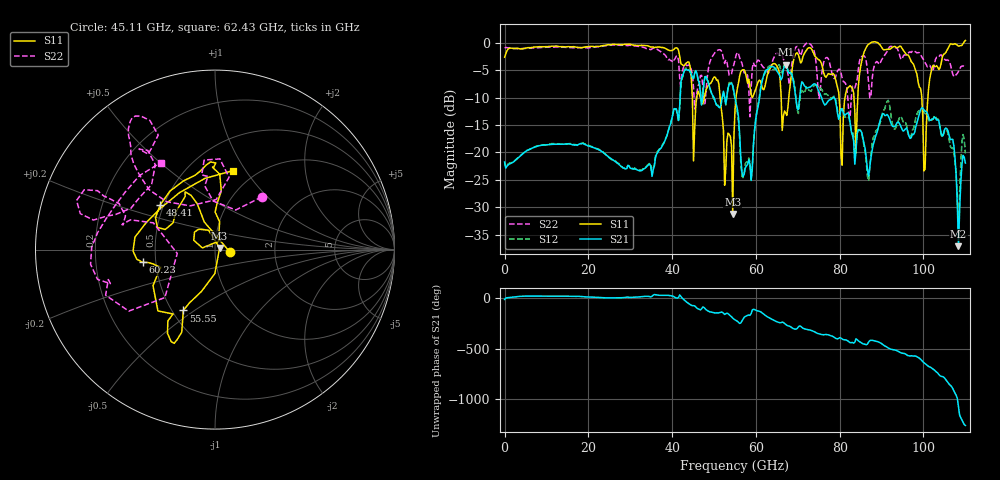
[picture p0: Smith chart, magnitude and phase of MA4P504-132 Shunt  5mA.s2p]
!Keysight Technologies,N5247B,US61255204,A.15.70.20
!Date: Friday, October 21, 2022 14:57:07
!Correction: S11(C  4-Port  )
!S31(C  4-Port  )
!S13(C  4-Port  )
!S33(C  4-Port  )
!S2P File: Measurements: S11, S31, S13, S33:
# Hz S  dB  R 50
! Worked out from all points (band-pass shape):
!   401 points, 10 MHz to 110 GHz, reference 50 ohm
!   highest |S21| = -3.97 dB at 67.1 GHz (marker M1); lowest = -37.1 dB at 108.4 GHz (marker M2)
!   |S21| within 3 dB of the highest: 42.14 GHz to 46.31 GHz (4.171 GHz wide, 9.43 % of centre); 61.5 GHz to 68.92 GHz (7.419 GHz wide, 11.4 % of centre)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
!   lowest |S11| = -31.2 dB at 54.46 GHz (marker M3), VSWR 1.06, Z = 52.6 + j0.972 ohm
!   |S11| at or under -10 dB: 51.47 GHz to 55.25 GHz (3.775 GHz wide, 7.07 % of centre); 66.03 GHz to 67.84 GHz (1.817 GHz wide, 2.71 % of centre); 79.85 GHz to 81.26 GHz (1.405 GHz wide, 1.74 % of centre)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
!   |S22| runs from -13.6 to 0.0 dB; largest |S21 - S12| = 0.24
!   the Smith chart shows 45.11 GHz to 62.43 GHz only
!   S11 on the Smith chart (normalised r, x): 45.11 GHz: 1.18, -0.03; 48.41 GHz: 0.48, +0.28; 55.55 GHz: 0.57, -0.45; 60.23 GHz: 0.42, -0.07; 62.43 GHz: 0.79, +0.88
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1e7  -2.61 -179.2  -21.76 -9.4  -21.74 -9.1  -0.92 -179.4
1.843332e10  -0.86 117.8  -18.36 18.7  -18.38 18.9  -0.87 124.4
3.685665e10  -0.75 115.3  -19.60 31.5  -19.46 31.4  -1.36 122.0
4.373102e10  -3.49 16.9  -4.98 -44.3  -4.82 -42.3  -4.10 80.8
4.51059e10  -21.56 -9.0  -6.50 -71.6  -6.51 -70.5  -8.12 48.4
4.84056e10  -8.09 140.8  -6.76 -121.5  -6.57 -121.0  -6.07 137.7
5.445505e10  -31.23 19.6  -7.80 164.5  -7.88 163.7  -4.62 160.5
5.5005e10  -12.23 -107.8  -10.02 146.4  -10.27 144.6  -3.14 166.3
5.555495e10  -8.35 -117.5  -12.04 133.0  -12.63 132.2  -1.74 160.5
5.72048e10  -4.91 -115.5  -23.98 172.3  -23.64 -177.2  -5.46 159.3
6.022952e10  -7.77 -170.0  -12.61 -122.4  -12.38 -117.7  -3.41 -165.8
6.242932e10  -6.91 77.2  -4.94 -175.1  -5.17 -168.7  -4.87 121.9
6.71039e10  -12.80 -41.6  -3.97 101.3  -3.65 101.7  -4.33 45.5
7.342832e10  -1.31 138.7  -7.73 37.6  -8.43 36.0  -0.68 108.5
8.112762e10  -10.62 -29.2  -13.21 -52.0  -13.52 -52.6  -7.17 -125.2
8.525225e10  -3.32 38.8  -16.33 -86.3  -16.41 -84.9  -2.46 -23.4
9.185165e10  -1.15 90.9  -13.81 -140.4  -11.16 -134.5  -0.77 83.7
9.872602e10  -7.19 150.4  -13.76 131.3  -12.54 130.9  -1.76 176.9
1.003759e11  -23.08 -28.6  -12.45 69.7  -12.90 71.6  -3.62 -155.7
1.036756e11  -4.87 -33.9  -14.25 -40.0  -14.14 -36.8  -2.55 -89.8
1.083502e11  -0.59 22.3  -37.12 0.0  -34.61 6.0  -5.19 -5.1
1.1e11  0.45 54.4  -21.94 172.1  -20.18 173.6  -4.09 16.6
